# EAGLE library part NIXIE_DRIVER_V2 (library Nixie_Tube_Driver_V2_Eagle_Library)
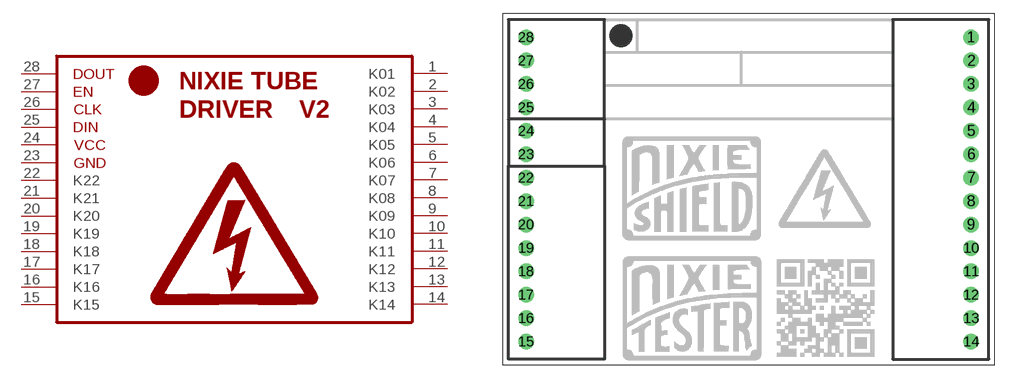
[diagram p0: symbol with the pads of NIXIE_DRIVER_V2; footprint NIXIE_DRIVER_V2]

Designator prefix -

## NIXIE_DRIVER_V2  [NIXIE_DRIVER_V2]
1  K01  pas
2  K02  pas
3  K03  pas
4  K04  pas
5  K05  pas
6  K06  pas
7  K07  pas
8  K08  pas
9  K09  pas
10  K10  pas
11  K11  pas
12  K12  pas
13  K13  pas
14  K14  pas
15  K15  pas
16  K16  pas
17  K17  pas
18  K18  pas
19  K19  pas
20  K20  pas
21  K21  pas
22  K22  pas
23  23  pwr
24  24  pwr
25  25  pas
26  26  pas
27  27  pas
28  28  pas

## Footprint NIXIE_DRIVER_V2 (pad centres in mm)
drill 1 pad 1.676: 1 22.86,17.78; 2 22.86,15.24; 3 22.86,12.7; 4 22.86,10.16; 5 22.86,7.62; 6 22.86,5.08; 7 22.86,2.54; 8 22.86,0; 9 22.86,-2.54; 10 22.86,-5.08; 11 22.86,-7.62; 12 22.86,-10.16; 13 22.86,-12.7; 14 22.86,-15.24; 15 -25.4,-15.24; 16 -25.4,-12.7; 17 -25.4,-10.16; 18 -25.4,-7.62; 19 -25.4,-5.08; 20 -25.4,-2.54; 21 -25.4,0; 22 -25.4,2.54; 23 -25.4,5.08; 24 -25.4,7.62; 25 -25.4,10.16; 26 -25.4,12.7; 27 -25.4,15.24; 28 -25.4,17.78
